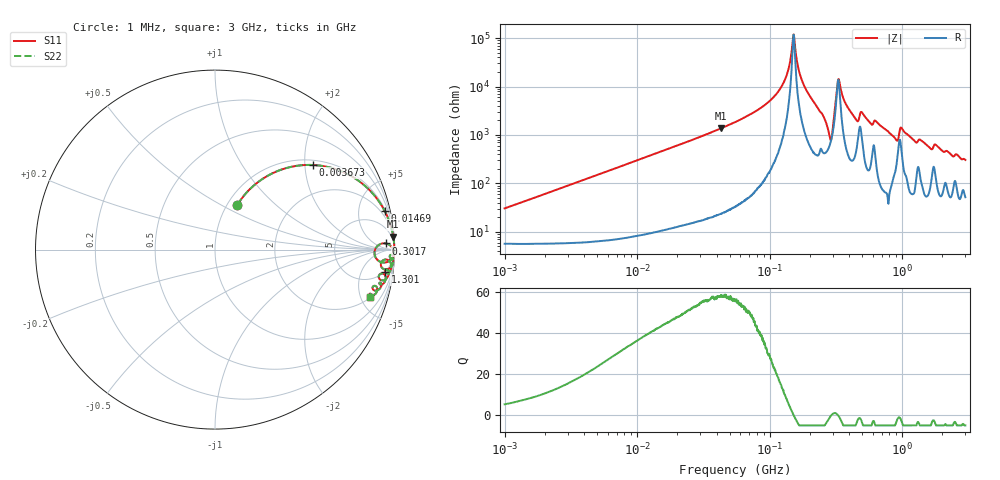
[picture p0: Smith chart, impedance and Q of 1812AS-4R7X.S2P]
!s-Parameter Generated by FASTRON Sdn. Bhd.
!FASTRON P/N : 1812AS-4R7X
!Keysight Technologies,E4991B,MY54100416,A.01.15
!Date created: Fri Oct 13 15:59:30 2023
!Version  : Rev00 Fri Oct 13 15:59:30 2023
!Data & Calibration Information:
!Freq	S11	S21	S12	S22
!PortZ  Port1:50+j0  Port2:50+j0
!When reading, reference impedance value at option line is always used.
! Remarks : This data is being provided solely for informational purposes.
# Hz S dB R 50
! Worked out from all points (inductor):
!   1601 points, 1 MHz to 3 GHz, reference 50 ohm
!   read as one part in series: L = 4.77 uH near 1.041 MHz
!   highest Q = 57.8 at 42.86 MHz (marker M1), where L = 5.07 uH
!   self-resonance near 151.3 MHz
!   S11 on the Smith chart (normalised r, x): 1 MHz: 1.11, +0.60; 3.673 MHz: 1.12, +2.20; 14.69 MHz: 1.21, +8.81; 301.7 MHz: 27, +20; 1.301 GHz: 5, -14; 3 GHz: 2.04, -6.01
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1000000  -11.12 63.4  -0.82 -15.9  -0.82 -15.9  -11.12 63.4
3673095  -2.84 40.8  -3.68 -46.1  -3.68 -46.1  -2.84 40.8
3804036  -2.70 39.9  -3.84 -47.0  -3.84 -47.0  -2.70 39.9
1.447069e7  -0.27 12.9  -13.01 -75.7  -13.01 -75.7  -0.27 12.9
1.468956e7  -0.26 12.7  -13.14 -75.9  -13.14 -75.9  -0.26 12.7
4.286213e7  -0.03 4.2  -22.74 -84.8  -22.74 -84.8  -0.03 4.2
5.477226e7  -0.02 3.1  -25.31 -85.9  -25.31 -85.9  -0.02 3.1
1.148668e8  -0.01 0.8  -37.59 -86.2  -37.59 -86.2  -0.01 0.8
1.341416e8  -0.01 0.3  -44.56 -82.5  -44.56 -82.5  -0.01 0.3
1.512587e8  -0.01 0.0  -61.44 -9.6  -61.44 -9.6  -0.01 0.0
1.731398e8  -0.01 -0.4  -43.32 81.0  -43.32 81.0  -0.01 -0.4
2.083556e8  -0.02 -1.0  -34.79 83.8  -34.79 83.8  -0.02 -1.0
2.841474e8  -0.65 -4.3  -19.80 42.8  -19.80 42.8  -0.65 -4.3
3.017325e8  -0.41 2.0  -24.72 -35.9  -24.72 -35.9  -0.41 2.0
3.220132e8  -0.09 0.3  -39.04 -28.8  -39.04 -28.8  -0.09 0.3
3.351655e8  -0.05 -0.3  -42.29 41.8  -42.29 41.8  -0.05 -0.3
4.480278e8  -0.10 -2.6  -26.53 75.3  -26.53 75.3  -0.10 -2.6
5.001674e8  -0.08 -1.9  -29.21 73.8  -29.21 73.8  -0.08 -1.9
7.925923e8  -0.06 -5.0  -21.19 82.8  -21.19 82.8  -0.06 -5.0
9.977393e8  -0.19 -4.0  -22.82 70.5  -22.82 70.5  -0.19 -4.0
1.300759e9  -0.39 -7.4  -17.44 67.1  -17.44 67.1  -0.39 -7.4
3e9  -0.86 -17.0  -10.54 63.2  -10.54 63.2  -0.86 -17.0
